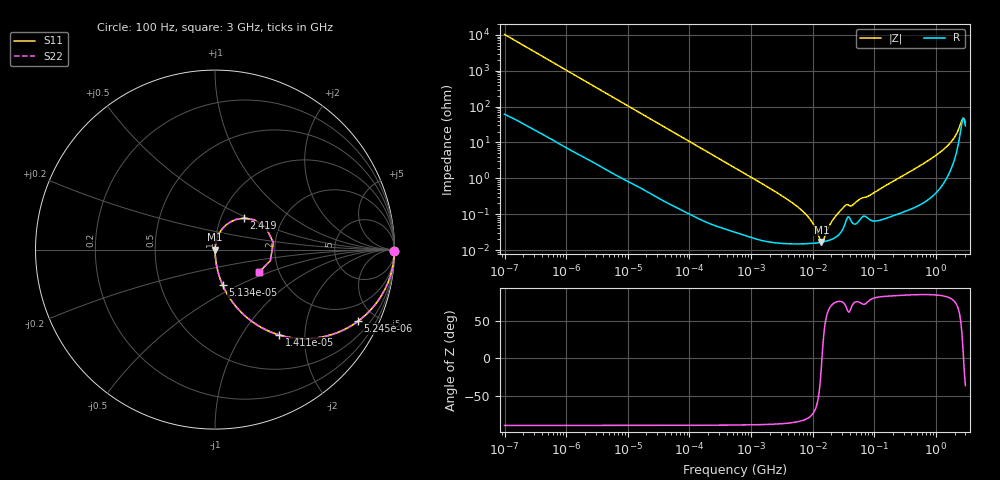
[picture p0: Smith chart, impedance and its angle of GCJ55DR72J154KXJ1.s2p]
!Murata Part Number: GCJ55DR72J154KXJ1
!These Parameters are Measured in Series Mode Connection
!Data Generated on Mar 13, 2026
!  o--ll--o
!Port1  Port2
!  o------o
!Operation Temp=25[degC], DC Bias Voltage=0[V]
!Freq. Start=100[Hz] Stop=3[GHz] 401[Steps]
# Hz S RI R 50
!Freq.(Hz) S11(Real) S11(Imag) S21(Real) S21(Imag) S12(Real) S12(Imag) S22(Real) S22(Imag)
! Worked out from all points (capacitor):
!   401 points, 100 Hz to 3 GHz, reference 50 ohm
!   read as one part in series: C = 154 nF near 109 Hz
!   lowest |Z| = 16.9 mohm at 13.82 MHz (marker M1)
!   series resonance near 14.12 MHz, so ESL is about 820 pH
!   S11 on the Smith chart (normalised r, x): 100 Hz: open; 5.245 kHz: 1.03, -4.00; 14.12 kHz: 1.01, -1.49; 51.34 kHz: 1.00, -0.41; 2.419 GHz: 1.28, +0.48; 3 GHz: 1.58, -0.43
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100  0.9998 -0.00971  0.000152 0.00971  0.000152 0.00971  0.9998 -0.00971
1788  0.9703 -0.1662  0.0297 0.1662  0.0297 0.1662  0.9703 -0.1662
5245  0.798 -0.3978  0.202 0.3978  0.202 0.3978  0.798 -0.3978
8791  0.5875 -0.4885  0.4125 0.4885  0.4125 0.4885  0.5875 -0.4885
14115  0.3587 -0.4756  0.6413 0.4756  0.6413 0.4756  0.3587 -0.4756
31977  0.1006 -0.2967  0.8994 0.2967  0.8994 0.2967  0.1006 -0.2967
51340  0.0425 -0.1974  0.9575 0.1974  0.9575 0.1974  0.0425 -0.1974
547723  0.000696 -0.0196  0.9993 0.0196  0.9993 0.0196  0.000696 -0.0196
4513443  0.000153 -0.00216  0.9998 0.00216  0.9998 0.00216  0.000153 -0.00216
7246509  0.00015 -0.0011  0.9998 0.0011  0.9998 0.0011  0.00015 -0.0011
9794414  0.000154 -0.000576  0.9998 0.000576  0.9998 0.000576  0.000154 -0.000576
1.382041e7  0.000165 -3.26e-05  0.9998 3.26e-05  0.9998 3.26e-05  0.000165 -3.26e-05
1.506283e7  0.00017 0.000101  0.9998 -0.000101  0.9998 -0.000101  0.00017 0.000101
2.12544e7  0.000206 0.000665  0.9998 -0.000665  0.9998 -0.000665  0.000206 0.000665
3.268714e7  0.000486 0.00159  0.9995 -0.00159  0.9995 -0.00159  0.000486 0.00159
4.418008e7  0.000568 0.0017  0.9994 -0.0017  0.9994 -0.0017  0.000568 0.0017
1.751444e8  0.000877 0.00715  0.9991 -0.00715  0.9991 -0.00715  0.000877 0.00715
1.163803e9  0.00801 0.0522  0.992 -0.0522  0.992 -0.0522  0.00801 0.0522
1.789813e9  0.0297 0.1008  0.9703 -0.1008  0.9703 -0.1008  0.0297 0.1008
2.419119e9  0.161 0.175  0.839 -0.175  0.839 -0.175  0.161 0.175
2.636591e9  0.2836 0.1241  0.7164 -0.1241  0.7164 -0.1241  0.2836 0.1241
3e9  0.2466 -0.1253  0.7534 0.1253  0.7534 0.1253  0.2466 -0.1253
